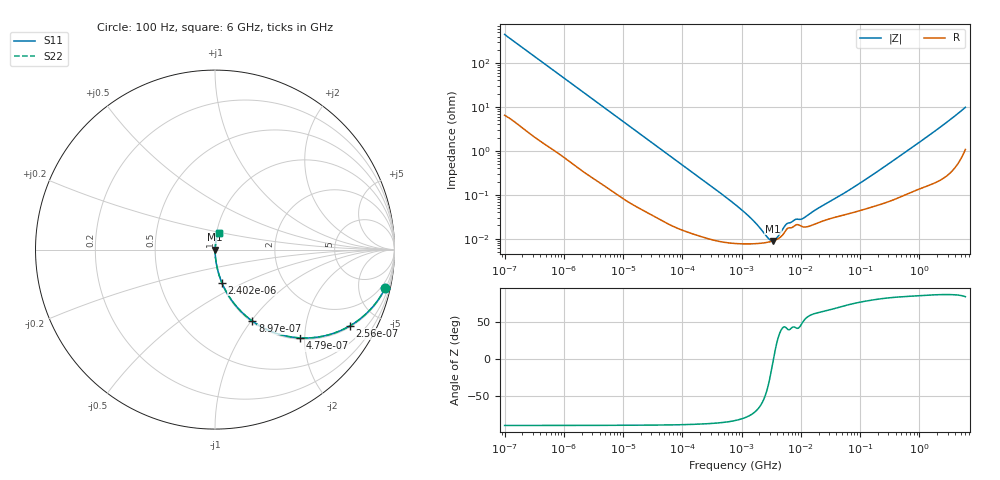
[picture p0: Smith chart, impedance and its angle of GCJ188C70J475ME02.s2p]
!Murata Part Number: GCJ188C70J475ME02
!These Parameters are Measured in Series Mode Connection
!Data Generated on Mar 13, 2026
!  o--ll--o
!Port1  Port2
!  o------o
!Operation Temp=25[degC], DC Bias Voltage=0[V]
!Freq. Start=100[Hz] Stop=6[GHz] 401[Steps]
# Hz S RI R 50
!Freq.(Hz) S11(Real) S11(Imag) S21(Real) S21(Imag) S12(Real) S12(Imag) S22(Real) S22(Imag)
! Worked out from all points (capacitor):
!   401 points, 100 Hz to 6 GHz, reference 50 ohm
!   read as one part in series: C = 3.56 uF near 109 Hz
!   lowest |Z| = 8.93 mohm at 3.394 MHz (marker M1)
!   series resonance near 3.456 MHz, so ESL is about 600 pH
!   S11 on the Smith chart (normalised r, x): 100 Hz: 1.13, -8.91; 256 Hz: 1.05, -3.51; 479 Hz: 1.03, -1.89; 897 Hz: 1.02, -1.02; 2.402 kHz: 1.01, -0.38; 6 GHz: 1.02, +0.19
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100  0.9492 -0.2124  0.0508 0.2124  0.0508 0.2124  0.9492 -0.2124
164  0.8786 -0.3191  0.1214 0.3191  0.1214 0.3191  0.8786 -0.3191
256  0.7523 -0.4245  0.2477 0.4245  0.2477 0.4245  0.7523 -0.4245
479  0.4717 -0.4918  0.5283 0.4918  0.5283 0.4918  0.4717 -0.4918
897  0.2085 -0.3986  0.7915 0.3986  0.7915 0.3986  0.2085 -0.3986
2008  0.0526 -0.2157  0.9474 0.2157  0.9474 0.2157  0.0526 -0.2157
2402  0.038 -0.1835  0.962 0.1835  0.962 0.1835  0.038 -0.1835
7358  0.00504 -0.0628  0.995 0.0628  0.995 0.0628  0.00504 -0.0628
40335  0.000417 -0.0117  0.9996 0.0117  0.9996 0.0117  0.000417 -0.0117
774597  7.8e-05 -0.0006  0.9999 0.0006  0.9999 0.0006  7.8e-05 -0.0006
1516199  7.65e-05 -0.000262  0.9999 0.000262  0.9999 0.000262  7.65e-05 -0.000262
2713602  8.26e-05 -7.03e-05  0.9999 7.03e-05  0.9999 7.03e-05  8.26e-05 -7.03e-05
3394479  8.91e-05 -5.2e-06  0.9999 5.2e-06  0.9999 5.2e-06  8.91e-05 -5.2e-06
4060267  9.87e-05 4.8e-05  0.9999 -4.8e-05  0.9999 -4.8e-05  9.87e-05 4.8e-05
5809218  0.000166 0.000144  0.9998 -0.000144  0.9998 -0.000144  0.000166 0.000144
7947587  0.000199 0.000183  0.9998 -0.000183  0.9998 -0.000183  0.000199 0.000183
1.087309e7  0.000186 0.000221  0.9998 -0.000221  0.9998 -0.000221  0.000186 0.000221
1.555665e7  0.000203 0.000349  0.9998 -0.000349  0.9998 -0.000349  0.000203 0.000349
7.129496e7  0.000385 0.00132  0.9996 -0.00132  0.9996 -0.00132  0.000385 0.00132
3.124326e8  0.000732 0.00515  0.9993 -0.00515  0.9993 -0.00515  0.000732 0.00515
1.95892e9  0.00283 0.0298  0.9972 -0.0298  0.9972 -0.0298  0.00283 0.0298
6e9  0.0197 0.0944  0.9803 -0.0944  0.9803 -0.0944  0.0197 0.0944
